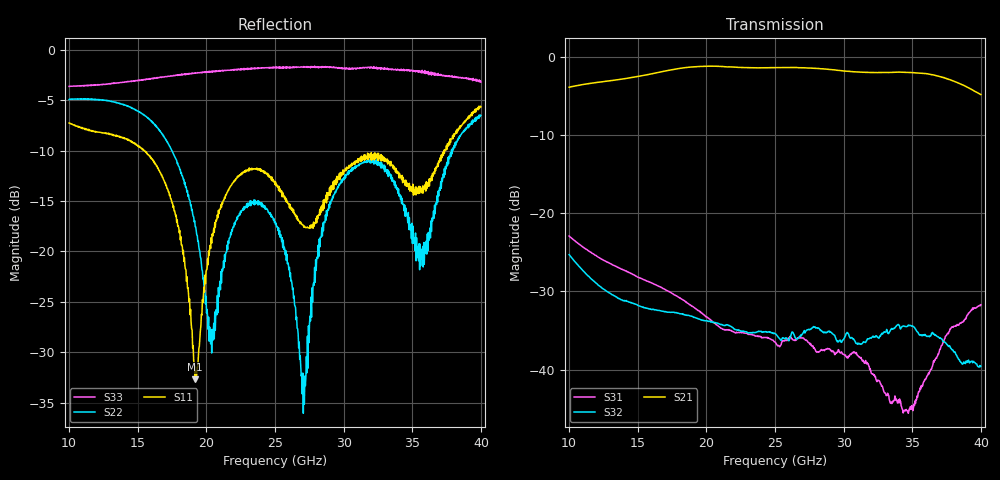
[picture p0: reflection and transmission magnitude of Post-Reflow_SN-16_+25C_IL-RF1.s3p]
!Agilent Technologies,N5245A,US49150155,A.09.90.19
!Agilent N5245A: A.09.90.19
!Date: Monday, November 12, 2018 23:21:20
!Correction: S11(Full 3 Port(1,2,3))
!S12(Full 3 Port(1,2,3))
!S13(Full 3 Port(1,2,3))
!S21(Full 3 Port(1,2,3))
!S22(Full 3 Port(1,2,3))
!S23(Full 3 Port(1,2,3))
!S31(Full 3 Port(1,2,3))
!S32(Full 3 Port(1,2,3))
!S33(Full 3 Port(1,2,3))
!S3P File: Measurements: <S11,S12,S13>,
!<S21,S22,S23>,
!<S31,S32,S33>:
# Hz S  dB  R 50
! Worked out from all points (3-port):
!   801 points, 10 GHz to 40 GHz, reference 50 ohm
!   strongest paths, dB at 10 GHz, 17.5 GHz, 25 GHz, 32.5 GHz, 40 GHz:
!     S21: -3.9, -1.6, -1.4, -2.0, -4.8
!     S32: -25.3, -32.7, -35.4, -35.9, -39.5
!     S31: -22.9, -30.2, -36.5, -41.3, -31.7
!   lowest |S11| = -32.7 dB at 19.19 GHz (marker M1), VSWR 1.05, Z = 47.8 - j0.289 ohm
!   |S11| at or under -10 dB: 15.46 GHz to 37.3 GHz (21.84 GHz wide, 82.8 % of centre); 37.30283 GHz to 37.36515 GHz (62.32 MHz wide, 0.167 % of centre)
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1e10  -7.27 8.3  -3.86 -159.2  -22.90 81.2
      -3.86 -159.0  -4.94 -105.0  -25.30 14.5
      -22.90 81.6  -25.28 14.6  -3.64 59.1
1.5175e10  -9.66 -145.3  -2.44 89.1  -28.28 -12.3
           -2.43 89.2  -6.20 160.9  -31.92 -77.7
           -28.29 -11.8  -31.89 -77.5  -3.02 -44.8
1.91875e10  -32.70 -172.5  -1.24 -1.2  -32.18 -86.8
            -1.24 -1.0  -17.56 89.3  -33.35 -161.7
            -32.16 -86.0  -33.35 -161.2  -2.29 -109.9
2.035e10  -18.64 -105.3  -1.18 -28.3  -33.74 -104.6
          -1.17 -28.1  -27.75 135.9  -33.95 173.0
          -33.71 -104.4  -33.92 173.3  -2.18 -126.7
2.5e10  -13.38 177.2  -1.36 -132.1  -36.49 -165.6
        -1.36 -132.0  -17.05 112.1  -35.39 66.0
        -36.49 -165.0  -35.41 66.8  -1.79 175.9
2.71e10  -17.61 176.4  -1.37 179.9  -36.02 160.3
         -1.37 -179.8  -32.42 -26.5  -35.23 26.0
         -36.00 160.6  -35.16 26.8  -1.67 151.4
3.085e10  -11.04 -178.0  -1.91 93.8  -37.92 98.3
          -1.90 94.3  -11.78 165.7  -36.59 -68.7
          -37.91 97.9  -36.43 -67.9  -1.83 106.6
3.4975e10  -13.60 146.4  -2.01 -4.5  -44.97 71.4
           -2.00 -4.0  -17.22 28.9  -34.45 -167.5
           -44.60 72.8  -34.45 -167.0  -2.08 47.5
3.74125e10  -9.92 164.6  -2.75 -68.9  -35.77 53.4
            -2.73 -68.8  -11.59 -151.6  -36.59 99.8
            -35.73 53.5  -36.53 100.6  -2.64 6.9
4e10  -5.66 119.1  -4.80 -136.3  -31.76 -15.8
      -4.81 -136.1  -6.52 128.6  -39.59 -43.5
      -31.70 -14.6  -39.55 -42.5  -3.19 -38.6
